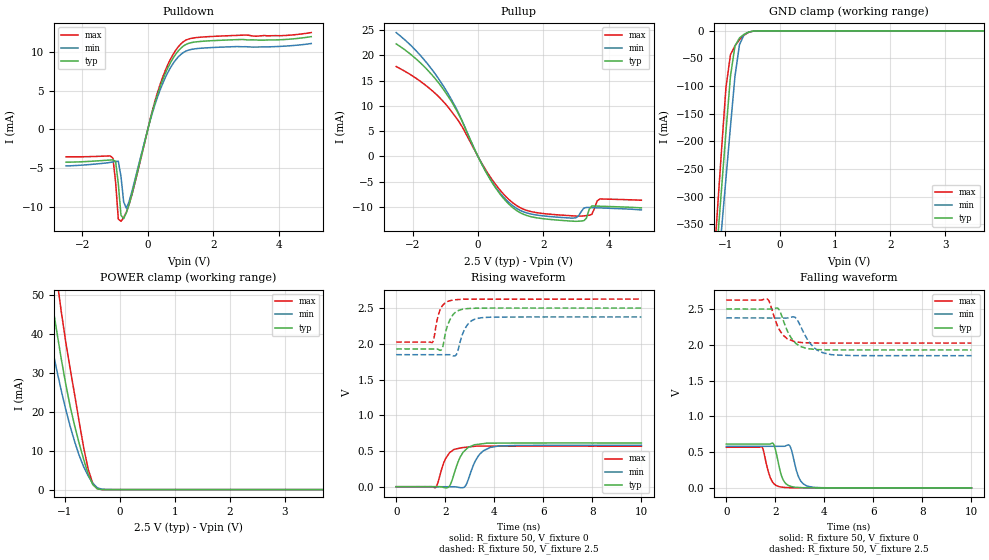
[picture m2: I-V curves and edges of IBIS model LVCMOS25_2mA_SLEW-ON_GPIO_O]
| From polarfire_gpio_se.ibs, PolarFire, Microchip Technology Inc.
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|   Model LVCMOS25_2mA_SLEW-ON_GPIO_O
[Model]   LVCMOS25_2mA_SLEW-ON_GPIO_O
Model_type   Output
Polarity   Non-Inverting
Enable   Active-High
Vmeas =   1.25
Cref =   5p
Rref =   1M
|   typ   min   max
C_comp_pullup   2.605e-12   2.605e-12   2.76e-12
C_comp_pulldown  2.605e-12   2.605e-12   2.76e-12
[Temperature Range]  25C   100C   -40C
[Voltage Range]  2.5   2.375   2.625
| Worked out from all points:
|   slope of the pulldown table from 0 to 0.375 V, typ, clamps not added: 68.5 ohm
|   slope of the pullup table from 0 to 0.375 V, typ, clamps not added: 82.3 ohm
|   GND clamp passes 1 mA (typ) near -0.51 V on its own axis
|   POWER clamp passes 1 mA (typ) near -0.47 V on its own axis
|   rising waveform, R_fixture 50, V_fixture 0: 20-80 % time 443ps typ, 478ps min, 385ps max; typ from 0 V to 0.612 V
|   rising waveform, R_fixture 50, V_fixture 2.5: 20-80 % time 323ps typ, 361ps min, 260ps max; typ from 1.93 V to 2.5 V
|   falling waveform, R_fixture 50, V_fixture 0: 20-80 % time 270ps typ, 297ps min, 275ps max; typ from 0.612 V to 0 V
|   falling waveform, R_fixture 50, V_fixture 2.5: 20-80 % time 498ps typ, 588ps min, 441ps max; typ from 2.5 V to 1.93 V
[GND Clamp]
| Voltage   I(typ)   I(min)   I(max)
-2.5V     -2.154A    -2.019A    -2.334A
-1.23V    -500.9mA   -550.5mA   -458.7mA
-1.148V   -394.9mA   -456.3mA   -338.7mA
-1.066V   -289mA     -362mA     -218.7mA
-984.4mV  -183.1mA   -267.7mA   -102.9mA
-902.3mV  -82.21mA   -173.6mA   -43.25mA
-820.3mV  -27.37mA   -82.26mA   -27.26mA
-738.3mV  -12.87mA   -24.95mA   -16.13mA
-656.2mV  -6.285mA   -7.324mA   -7.886mA
-574.2mV  -2.342mA   -2.429mA   -2.872mA
-328.1mV  -3.985uA   -10.42uA   -2.675uA
5V        0A         0A         0A
[POWER Clamp]
| Voltage   I(typ)   I(min)   I(max)
-2.5V     191.3mA    155.6mA    232.6mA
-1.559V   79.6mA     61.42mA    102.5mA
-1.395V   63.37mA    48.38mA    82.85mA
-1.23V    48.04mA    36.4mA     63.67mA
-1.148V   40.77mA    30.8mA     54.53mA
-1.066V   33.71mA    25.51mA    45.88mA
-820.3mV  16.31mA    12.25mA    24.25mA
-656.2mV  7.665mA    5.818mA    10.67mA
-574.2mV  3.929mA    3.48mA     5.131mA
-492.2mV  1.272mA    1.622mA    1.634mA
-410.2mV  189.8uA    467.6uA    244.4uA
5V        0A         0A         0A
[Pullup]
| Voltage   I(typ)   I(min)   I(max)
-2.5V     22.26mA    24.49mA    17.77mA
-1.066V   13.35mA    14.01mA    10.89mA
-492.2mV  7.057mA    7.171mA    5.969mA
312.5mV   -3.874mA   -3.789mA   -3.432mA
1.094V    -10.29mA   -9.9mA     -9.323mA
2.344V    -12.55mA   -11.98mA   -11.52mA
2.992V    -12.84mA   -12.16mA   -11.8mA
3.156V    -12.8mA    -10.96mA   -11.81mA
3.32V     -12.22mA   -10.1mA    -11.71mA
3.484V    -9.804mA   -10.14mA   -11.46mA
3.73V     -9.86mA    -10.2mA    -8.423mA
5V        -10.2mA    -10.59mA   -8.676mA
[Pulldown]
| Voltage   I(typ)   I(min)   I(max)
-2.5V     -4.252mA   -4.738mA   -3.553mA
-1.066V   -3.946mA   -4.218mA   -3.737mA
-984.4mV  -4.157mA   -4.155mA   -6.85mA
-902.3mV  -7.055mA   -4.125mA   -11.6mA
-820.3mV  -11.11mA   -6.095mA   -11.89mA
-738.3mV  -11.55mA   -9.39mA    -11.41mA
-656.2mV  -10.78mA   -10.21mA   -10.71mA
312.5mV   4.706mA    4.352mA    4.968mA
625mV     8.048mA    7.446mA    8.475mA
1.016V    10.51mA    9.701mA    11.07mA
1.562V    11.34mA    10.46mA    11.89mA
5V        11.98mA    11.09mA    12.51mA
[Ramp]
dV/dt_r   0.367135/0.443285n  0.348077/0.477899n  0.340496/0.385274n
dV/dt_f   0.343513/0.497822n  0.316364/0.588486n  0.360573/0.441093n
R_load = 50
[Rising Waveform]
R_fixture = 50
V_fixture = 0
V_fixture_min = 0
V_fixture_max = 0
| Time   V(typ)   V(min)   V(max)
0s        25.93nV    47.05nV    33.34nV
1.603ns   875.1uV    -368.8uV   -13.28mV
1.938ns   -10.62mV   -445.9uV   333.6mV
2.129ns   -7.727mV   -489.9uV   451.8mV
2.237ns   51.19mV    -514.7uV   492.2mV
2.656ns   440.8mV    -14.02mV   544.9mV
2.843ns   519.9mV    20.75mV    552mV
3.333ns   593.1mV    421.8mV    568mV
3.833ns   609.5mV    549.5mV    567.9mV
10ns      611.9mV    580.1mV    567.5mV
[Rising Waveform]
R_fixture = 50
V_fixture = 2.5
V_fixture_min = 2.375
V_fixture_max = 2.625
| Time   V(typ)   V(min)   V(max)
0s        1.927V     1.848V     2.024V
1.472ns   1.927V     1.848V     2.019V
1.819ns   1.909V     1.848V     2.496V
1.902ns   1.962V     1.848V     2.541V
2.09ns    2.25V      1.848V     2.591V
2.322ns   2.409V     1.832V     2.614V
2.485ns   2.457V     1.871V     2.618V
2.875ns   2.491V     2.251V     2.624V
3.386ns   2.499V     2.36V      2.624V
10ns      2.5V       2.375V     2.625V
[Falling Waveform]
R_fixture = 50
V_fixture = 0
V_fixture_min = 0
V_fixture_max = 0
| Time   V(typ)   V(min)   V(max)
0s        611.9mV    580.2mV    567.5mV
1.446ns   611.9mV    580.5mV    573.5mV
1.769ns   612.8mV    580.5mV    166.1mV
1.902ns   621.8mV    580.6mV    72.94mV
2.31ns    117.4mV    580.7mV    8.517mV
2.54ns    32.18mV    600mV      2.881mV
2.648ns   18.5mV     536.9mV    1.957mV
2.974ns   4.862mV    132.4mV    100.1uV
3.36ns    1.111mV    19.36mV    94.62uV
10ns      1.268uV    4.431uV    625.2nV
[Falling Waveform]
R_fixture = 50
V_fixture = 2.5
V_fixture_min = 2.375
V_fixture_max = 2.625
| Time   V(typ)   V(min)   V(max)
0s        2.5V       2.375V     2.625V
1.679ns   2.499V     2.374V     2.637V
1.806ns   2.499V     2.374V     2.553V
2.1ns     2.51V      2.374V     2.253V
2.487ns   2.197V     2.374V     2.083V
2.813ns   2.027V     2.381V     2.041V
3.302ns   1.947V     2.077V     2.028V
3.585ns   1.936V     1.958V     2.026V
4.292ns   1.928V     1.861V     2.024V
10ns      1.927V     1.848V     2.024V
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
